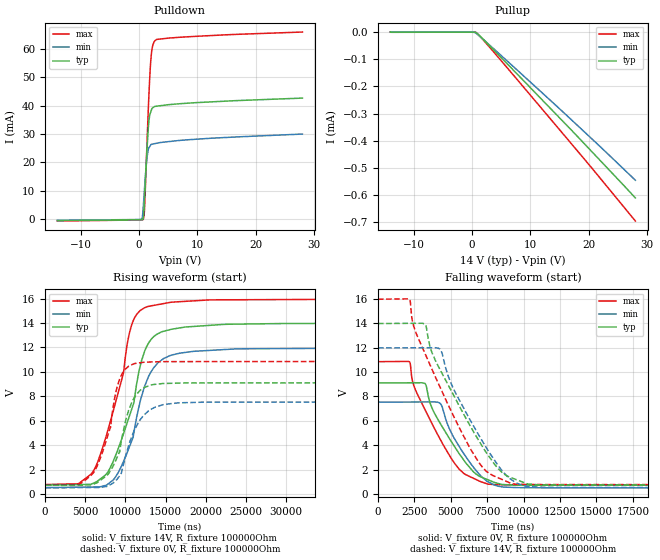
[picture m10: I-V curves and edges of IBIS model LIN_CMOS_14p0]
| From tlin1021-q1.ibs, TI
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|   LIN_CMOS_14p0
[Model]   LIN_CMOS_14p0
Model_type   Output
Polarity   Non-Inverting
Vmeas = 7
Vref = 7
Cref = 2pF
Rref = 100000
|   typ   min   max
C_comp   12.71pF   11.59pF   13.31pF
[Voltage Range]   14   12   16
[Temperature Range]   25   165   -55
[Pullup Reference]   14   12   16
[Pulldown Reference]   0   0   0
[Power Clamp Reference]   14   12   16
[GND Clamp Reference]   0   0   0
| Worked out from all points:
|   slope of the pulldown table from 0 to 2.1 V, typ, clamps not added: 54.3 ohm
|   slope of the pullup table from 0 to 2.1 V, typ, clamps not added: 70.8 kohm
|   falling waveform, V_fixture 0V, R_fixture 100000Ohm: 20-80 % time 2.56us typ, 2.09us min, 2.64us max; typ from 9.11 V to 0.708 V
|   rising waveform, V_fixture 14V, R_fixture 100000Ohm: 20-80 % time 3.3us typ, 3.08us min, 3.24us max; typ from 0.724 V to 14 V
|   rising waveform, V_fixture 0V, R_fixture 100000Ohm: 20-80 % time 2.21us typ, 2.33us min, 2.23us max; typ from 0.708 V to 9.11 V
|   falling waveform, V_fixture 14V, R_fixture 100000Ohm: 20-80 % time 3.64us typ, 3.16us min, 3.59us max; typ from 14 V to 0.724 V
[Pulldown]
|   Voltage   I(typ)   I(min)   I(max)
-14V      -610.8uA   -504.3uA   -748.2uA
214mV     -269.5uA   -217.8uA   -375.7uA
515.6mV   -240.6uA   84.63uA    -365uA
723.4mV   372.5uA    4.177mA    -114.6uA
778.4mV   1.041mA    5.813mA    314.5uA
923.8mV   6.295mA    10.14mA    2.846mA
1.387V    25.44mA    21.94mA    27.95mA
1.642V    33.44mA    24.9mA     41.34mA
1.953V    37.48mA    25.95mA    54.18mA
2.245V    39.07mA    26.43mA    60.35mA
2.786V    39.79mA    26.65mA    63.1mA
28V       42.71mA    29.99mA    66.06mA
[Pullup]
|   Voltage   I(typ)   I(min)   I(max)
-14V      376.4nA    334.9nA    525.4nA
214mV     -368.2nA   -195.9nA   -203.3nA
685.5mV   -1.181uA   -3.812uA   -1.079uA
2.16V     -31.16uA   -31.02uA   -34.2uA
8.71V     -175.7uA   -158.5uA   -199.1uA
20.28V    -434.4uA   -387.8uA   -493.9uA
28V       -610.9uA   -545.6uA   -695.9uA
[Ramp]
R_load = 100000
|   typ   min   max
dV/dt_r   7.95411/3.27602e-06   6.87685/3.06834e-06   9.1242/3.2325e-06
dV/dt_f   5.03837/2.54792e-06   4.22237/2.0893e-06   6.06486/2.6411e-06
[Falling Waveform]
V_fixture = 0V
V_fixture_min = 0V
V_fixture_max = 0V
R_fixture = 100000Ohm
C_fixture = 0F
|   Time   V(typ)   V(min)   V(max)
0s        9.105V     7.536V     10.85V
2.167us   9.117V     7.542V     10.84V
2.449us   9.119V     7.543V     8.91V
3.221us   9.067V     7.545V     6.925V
3.615us   7.325V     7.546V     5.99V
4.24us    5.854V     7.458V     4.551V
5.552us   3.343V     3.939V     2.062V
7.538us   1.164V     1.01V      806.9mV
9.639us   722.1mV    516.5mV    746.4mV
50us      708.2mV    499mV      743.5mV
[Rising Waveform]
V_fixture = 14V
V_fixture_min = 12V
V_fixture_max = 16V
R_fixture = 100000Ohm
C_fixture = 0F
|   Time   V(typ)   V(min)   V(max)
0s        724.4mV    520.4mV    767.7mV
4.157us   768.4mV    552.5mV    835.2mV
6.184us   928.1mV    568.2mV    2.069V
7.886us   1.87V      838.3mV    5.379V
9.525us   4.483V     2.299V     9.334V
10.74us   6.856V     4.271V     13.77V
12.38us   11.67V     8.797V     15.24V
14.78us   13.33V     11.1V      15.59V
18.49us   13.72V     11.68V     15.81V
50us      13.98V     11.98V     15.97V
[Rising Waveform]
V_fixture = 0V
V_fixture_min = 0V
V_fixture_max = 0V
R_fixture = 100000Ohm
C_fixture = 0F
|   Time   V(typ)   V(min)   V(max)
0s        708.2mV    499mV      743.5mV
4.239us   715.9mV    519mV      801.1mV
6.008us   799.5mV    527.4mV    1.725V
8.151us   1.925V     771.3mV    5.471V
8.68us    2.578V     1.017V     7.914V
9.457us   4.173V     1.619V     9.668V
11us      7.76V      5.04V      10.65V
13.02us   8.88V      6.868V     10.8V
16.61us   9.075V     7.461V     10.84V
50us      9.105V     7.536V     10.85V
[Falling Waveform]
|Gnd
V_fixture = 14V
V_fixture_min = 12V
V_fixture_max = 16V
R_fixture = 100000Ohm
C_fixture = 0F
|   Time   V(typ)   V(min)   V(max)
0s        13.98V     11.98V     15.97V
2.17us    14V        11.99V     15.97V
2.449us   14V        11.99V     13.75V
3.231us   13.93V     11.99V     11.51V
3.615us   11.91V     12V        10.48V
4.253us   10.22V     11.88V     8.781V
5.218us   8.037V     8.544V     6.32V
7.025us   4.173V     4.606V     2.421V
9.132us   1.342V     1.192V     864mV
50us      724.4mV    520.4mV    767.7mV
